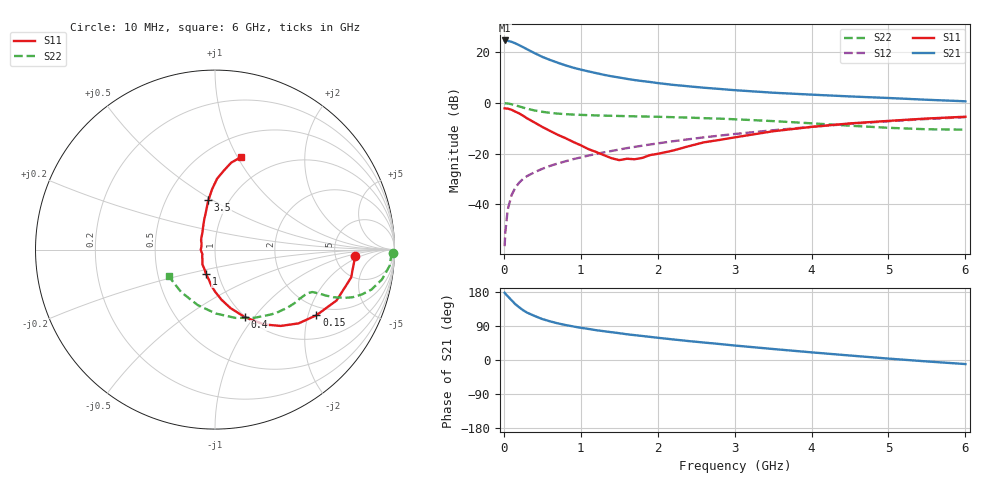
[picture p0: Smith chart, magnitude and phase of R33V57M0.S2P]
! SIEMENS Small Signal Semiconductors
! BFR181
! Si NPN RF Bipolar Junction Transistor in SOT23
! VCE = 3.5 V  IC = 7 mA
! Common Emitter S-Parameters:  May  1996
# GHz  S  MA  R  50
!  f  S11  S21  S12  S22
! GHz  MAG  ANG  MAG  ANG  MAG  ANG  MAG  ANG
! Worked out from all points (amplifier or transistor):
!   36 points, 10 MHz to 6 GHz, reference 50 ohm
!   highest |S21| = 24.6 dB at 10 MHz (marker M1)
!   |S21| within 3 dB of that: start of sweep to 272.4 MHz
!   unconditionally stable (mu >= 1): 946.3 MHz to 2.785 GHz
!   at 250 MHz: K = 0.50, MSG = 26.0 dB, |S12| = -29.9 dB
!   at 1.4 GHz: K = 1.06, MAG = 13.3 dB, |S12| = -18.9 dB
!   at 6 GHz: K = 0.86, MSG = 3.1 dB, |S12| = -5.6 dB
!   S11 on the Smith chart (normalised r, x): 10 MHz: 7.98, -1.41; 150 MHz: 1.69, -2.27; 400 MHz: 0.99, -0.90; 1 GHz: 0.87, -0.25; 3.5 GHz: 0.80, +0.48; 6 GHz: 0.72, +1.03
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0.01  0.7833 -2.5  17.08 177.4  0.0015 84.4  0.9897 -1.0
0.02  0.7788 -4.6  17.06 174.9  0.0029 84.7  0.9823 -2.2
0.05  0.7743 -11.6  16.81 168.3  0.0078 84.5  0.9773 -5.3
0.1  0.7343 -22.7  16.07 157.8  0.0152 79.4  0.9452 -10.1
0.15  0.6731 -32.9  14.97 147.1  0.0215 74.3  0.9001 -14.3
0.2  0.6213 -41.4  13.78 139.0  0.0269 71.7  0.8554 -17.0
0.25  0.561 -49.3  12.6 131.5  0.0319 69.0  0.8113 -19.1
0.3  0.4998 -56.6  11.49 125.2  0.036 68.2  0.7715 -20.4
0.4  0.4113 -66.2  9.607 116.2  0.0432 66.4  0.711 -21.9
0.5  0.3369 -75.2  8.11 108.1  0.0503 65.9  0.6694 -22.5
0.6  0.2811 -82.7  7.061 102.0  0.0573 65.8  0.6387 -22.8
0.7  0.2359 -89.6  6.224 96.8  0.064 66.3  0.6171 -23.1
0.8  0.2029 -95.7  5.527 92.4  0.0706 66.4  0.6019 -23.3
1  0.1463 -109.9  4.55 85.0  0.0844 67.1  0.5824 -24.2
1.1  0.123 -118.7  4.19 82.0  0.0917 67.3  0.5745 -24.9
1.3  0.0935 -138.1  3.591 76.0  0.1062 67.2  0.5625 -26.3
1.6  0.0794 -178.7  2.985 67.9  0.1287 66.7  0.5495 -29.2
2.2  0.1153 127.9  2.276 54.3  0.1759 64.2  0.5244 -36.6
3.5  0.2768 97.8  1.593 29.0  0.2901 54.4  0.4389 -60.0
4.5  0.3954 88.3  1.345 11.8  0.3873 43.8  0.3561 -89.3
5.5  0.4934 79.4  1.156 -3.8  0.4826 31.1  0.3028 -128.4
6  0.5351 74.3  1.079 -10.7  0.5251 24.1  0.2977 -150.1
